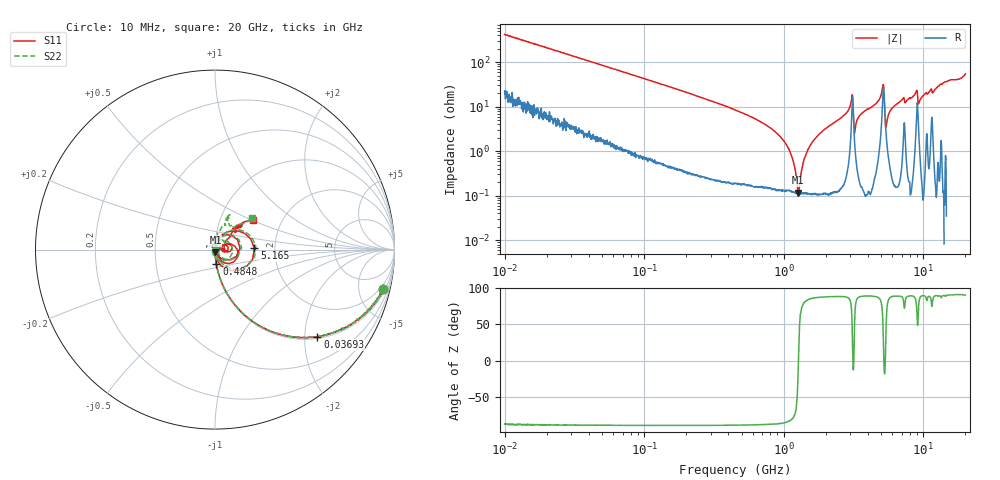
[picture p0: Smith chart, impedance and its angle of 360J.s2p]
!Keysight Technologies,P5008B,MY61100088,A.16.20.02
!Date: Tuesday, November 07, 2023 16:07:35
!Correction: S11(C  2-Port  )
!S21(C  2-Port  )
!S12(C  2-Port  )
!S22(C  2-Port  )
!S2P File: Measurements: S11, S21, S12, S22:Log Frequency Sweep
# Hz S  dB  R 50
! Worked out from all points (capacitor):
!   1601 points, 10 MHz to 20 GHz, reference 50 ohm
!   read as one part in series: C = 37.9 pF near 10.39 MHz
!   lowest |Z| = 116 mohm at 1.272 GHz (marker M1)
!   series resonance near 1.272 GHz, so ESL is about 410 pH
!   S11 on the Smith chart (normalised r, x): 10 MHz: 1.43, -8.36; 36.93 MHz: 1.04, -2.31; 484.8 MHz: 1.00, -0.17; 5.165 GHz: 1.56, +0.02; 20 GHz: 1.42, +0.51
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1e7  -0.34 -13.3  -12.79 73.7  -12.79 73.8  -0.34 -13.2
3.555162e7  -2.41 -39.5  -3.94 49.2  -3.94 49.2  -2.41 -39.5
3.692874e7  -2.50 -40.5  -3.76 48.5  -3.76 48.5  -2.50 -40.5
1.263918e8  -9.91 -70.7  -0.51 18.4  -0.51 18.4  -9.91 -70.6
4.472136e8  -20.87 -84.4  -0.05 4.5  -0.05 4.5  -20.86 -84.1
4.848288e8  -21.67 -84.9  -0.04 4.0  -0.05 4.0  -21.66 -84.5
1.271764e9  -36.18 -81.9  -0.01 -0.9  -0.01 -0.9  -36.19 -91.2
1.589917e9  -46.08 -56.8  -0.01 -2.0  -0.01 -2.0  -47.03 -98.9
1.765077e9  -49.29 9.8  -0.01 -2.6  -0.01 -2.6  -60.52 158.2
1.97824e9  -42.89 63.0  -0.01 -3.3  -0.01 -3.3  -44.43 89.2
3.048071e9  -20.54 58.3  -0.37 -9.8  -0.37 -9.8  -20.28 54.6
3.383874e9  -41.27 98.8  -0.02 -5.7  -0.03 -5.7  -38.47 32.0
3.651107e9  -32.60 94.0  -0.01 -7.0  -0.01 -7.0  -32.59 62.0
5.164568e9  -13.16 1.8  -2.09 -12.8  -2.09 -12.8  -12.84 5.5
5.652411e9  -32.32 -78.5  -0.04 -9.1  -0.04 -9.1  -33.54 -78.1
6.041124e9  -39.48 -21.3  0.00 -11.1  -0.00 -11.1  -52.55 145.8
6.999632e9  -27.68 29.0  -0.02 -14.6  -0.02 -14.6  -29.41 100.7
7.588373e9  -27.74 5.0  -0.01 -14.9  -0.02 -14.9  -31.76 129.6
9.003717e9  -17.94 -2.1  -0.86 -20.9  -0.86 -20.8  -20.35 12.6
9.901129e9  -32.90 -10.0  0.03 -20.1  0.02 -20.0  -37.32 146.2
1.361179e10  -16.25 44.9  -0.10 -29.1  -0.10 -29.0  -16.26 69.3
2e10  -11.42 38.4  -0.34 -51.7  -0.34 -51.5  -11.31 40.8
